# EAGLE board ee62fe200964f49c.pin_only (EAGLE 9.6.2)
REV: C

Size 25.4 x 22.86 mm. Coordinates in mm from the lower left corner, seen from the top.
Outline: 0,20.32 0,2.54 arc90 2.54,0 22.86,0 arc90 25.4,2.54 25.4,20.32 arc90 22.86,22.86 2.54,22.86 arc90 0,20.32
Copper layers (1*16): Top 0.035mm / dielectric 1.5mm / Bottom 0.035mm
Design rules "adafruit *": minimum track width 8mil, minimum drill 15.5mil, track to track 8mil, track to pad 8mil, pad to pad 8mil, via to via 8mil, smd to smd 8mil, copper to edge 10mil, drill to drill 8mil, minimum pad ring 10mil, minimum via ring 8mil, stop-mask expansion 2mil, vias tented up to drill 20mil, thermal gap 10mil
Net classes: 1 highpower: width 0.406 mm, drill 0.483 mm; 2 lowpower: width 0.254 mm, drill 0.381 mm

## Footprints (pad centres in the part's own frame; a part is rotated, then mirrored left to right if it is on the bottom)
0603-NO = smd 1.075 x 1: 1 -0.85,0; 2 0.85,0
0805-NO = smd 1.24 x 1.5: 1 -0.95,0; 2 0.95,0
JST_SH4 = smd 0.6 x 1.55: 1 -1.5,2.514; 2 -0.5,2.514; 3 0.5,2.514; 4 1.5,2.514 | smd 1.2 x 1.8: MT1 -2.8,-1.386; MT2 2.8,-1.386
CHIPLED_0603_NOOUTLINE = smd 0.8 x 0.8: A 0,-0.75; C 0,0.75
FIDUCIAL_1MM = smd 1 x 1: 1 0,0
1X06_ROUND_70 = drill 1 pad 1.778: 1 -6.35,0; 2 -3.81,0; 3 -1.27,0; 4 1.27,0; 5 3.81,0; 6 6.35,0
SOT363 = smd 0.5 x 0.5: 1 -0.75,-0.9; 3 0.75,-0.9; 4 0.75,0.9; 6 -0.75,0.9 | smd 0.4 x 0.5: 2 0,-0.9; 5 0,0.9
RESPACK_4X0603 = smd 0.45 x 0.9: 1 -1.3,-0.85; 2 -0.4,-0.85; 3 0.4,-0.85; 4 1.3,-0.85; 5 1.3,0.85; 6 0.4,0.85; 7 -0.4,0.85; 8 -1.3,0.85
SOLDERJUMPER_ARROW_NOPASTE = smd 0.762 x 1.524: 1 -1.016,0; 2 1.016,0
BNO080 = smd 0.25 x 0.675: 1 -2.25,1.562; 6 -2.25,-1.562; 7 -1.75,-1.562; 8 -1.25,-1.562; 9 -0.75,-1.562; 10 -0.25,-1.562; 11 0.25,-1.562; 12 0.75,-1.562; 13 1.25,-1.562; 14 1.75,-1.562; 15 2.25,-1.562; 20 2.25,1.562; 21 1.75,1.562; 22 1.25,1.562; 23 0.75,1.562; 24 0.25,1.562; 25 -0.25,1.562; 26 -0.75,1.562; 27 -1.25,1.562; 28 -1.75,1.562 | smd 0.575 x 0.25: 2 -2.312,0.75; 3 -2.312,0.25; 4 -2.312,-0.25; 5 -2.312,-0.75; 16 2.312,-0.75; 17 2.312,-0.25; 18 2.312,0.25; 19 2.312,0.75
SOT23-5 = smd 0.55 x 1.2: 1 -0.95,-1.3; 2 0,-1.3; 3 0.95,-1.3; 4 0.95,1.3; 5 -0.95,1.3
TSSOP16 = smd 0.305 x 0.991: 1 -2.275,-2.918; 2 -1.625,-2.918; 3 -0.975,-2.918; 4 -0.325,-2.918; 5 0.325,-2.918; 6 0.975,-2.918; 7 1.625,-2.918; 8 2.275,-2.918; 9 2.275,2.918; 10 1.625,2.918; 11 0.975,2.918; 12 0.325,2.918; 13 -0.325,2.918; 14 -0.975,2.918; 15 -1.625,2.918; 16 -2.275,2.918
MOUNTINGHOLE_2.5_PLATED = drill 2.5 pad 3.2: P$1 0,0
XTAL3215 = smd 1.1 x 1.9: P$1 1.2,0; P$2 -1.2,0

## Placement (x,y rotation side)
C1  0.1uF  [0603-NO]  7.49,13.72 180 top
C2  10uF  [0805-NO]  3.05,6.54 270 top
C3  10uF  [0805-NO]  6.92,9.78 90 top
C4  0.1uF  [0603-NO]  7.68,12.38 0 top
C5  0.1uF  [0603-NO]  24.19,16.57 270 top
C6  22pF  [0603-NO]  8.76,16.13 90 top
C7  22pF  [0603-NO]  14.1,15.88 270 top
CONN3  STEMMA_I2C_QT  [JST_SH4]  22.86,11.43 90 top
CONN4  STEMMA_I2C_QT  [JST_SH4]  2.54,11.43 270 top
D1  GREEN  [CHIPLED_0603_NOOUTLINE]  1.52,15.49 90 top
FID3  FIDUCIAL_1MM  [FIDUCIAL_1MM]  1.08,17.65 0 top
FID4  FIDUCIAL_1MM  [FIDUCIAL_1MM]  19.43,7.49 0 top
JP1  [1X06_ROUND_70]  12.7,2.54 0 top
JP2  [1X06_ROUND_70]  12.7,20.32 0 top
Q2  BSS138  [SOT363]  21.59,16 0 top
R2  10K  [RESPACK_4X0603]  6.03,16.26 180 top
R3  10K  [RESPACK_4X0603]  18.22,15.81 0 top
R4  10K  [RESPACK_4X0603]  17.97,11.62 90 top
SJ1  PS1  [SOLDERJUMPER_ARROW_NOPASTE]  10.99,16.76 180 bottom
SJ2  PS0  [SOLDERJUMPER_ARROW_NOPASTE]  7.62,16.76 0 bottom
U1  BNO080  [BNO080]  12.7,12.26 0 top
U2  AP2112K-3.3  [SOT23-5]  6.03,6.22 270 top
U3  74AHC4050  [TSSOP16]  12.19,7.37 270 top
U$1  MOUNTINGHOLE2.5  [MOUNTINGHOLE_2.5_PLATED]  2.54,20.32 0 top
U$17  MOUNTINGHOLE2.5  [MOUNTINGHOLE_2.5_PLATED]  22.86,20.32 0 top
U$19  MOUNTINGHOLE2.5  [MOUNTINGHOLE_2.5_PLATED]  2.54,2.54 0 top
U$21  MOUNTINGHOLE2.5  [MOUNTINGHOLE_2.5_PLATED]  22.86,2.54 0 top
U$22  [ADAFRUIT_3.5MM]  24.13,4.45 90 top
U$25  [PCBFEAT-REV-040]  1.45,17.37 0 bottom
U$30  [STEMMAQT]  22.61,6.99 90 bottom
U$31  [STEMMAQT]  2.79,15.88 270 bottom
X1  32.768  [XTAL3215]  11.43,16.32 180 top

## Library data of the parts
C1-C7 CONN3 CONN4 D1 JP1 JP2 Q2 R2-R4 U1-U3 U$22 U$25 = microbuilder
FID3 FID4 SJ1 SJ2 U$1 U$17 U$19 U$21 = microbuilder; BOM: EXCLUDE
U$30 U$31 = silks
X1 = adafruit2

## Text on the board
tPlace: BT | P0 | P1 | RST | DI | CS | BNO08x 9-DoF | on | Y | X | Z | 3Vo | SCL | VIN | GND | SDA | INT
bPlace: PS0 | PS1 | BNO08x 9-DoF | Adv. Inertial / Measurement Unit / 9DoF Accel/Gyro/Mag / Quat. & Euler output / I2C/UART/SPI Interface | VLogic/Vcc: 3-5VDC

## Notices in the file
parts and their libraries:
microbuilder: This work is placed in the public domain, and may be freely used for commercial and non-commercial work with the following conditions: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
